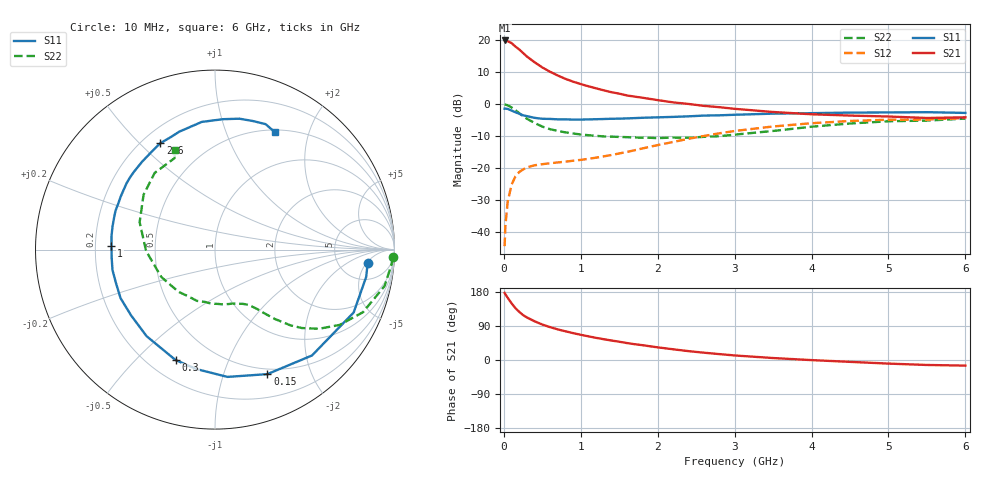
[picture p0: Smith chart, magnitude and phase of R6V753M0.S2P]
! SIEMENS Small Signal Semiconductors
! BFR193
! Si NPN RF Bipolar Junction Transistor in SOT23
! VCE = 0.75 V  IC = 3 mA
! Common Emitter S-Parameters:  May  1996
# GHz  S  MA  R  50
!  f  S11  S21  S12  S22
! GHz  MAG  ANG  MAG  ANG  MAG  ANG  MAG  ANG
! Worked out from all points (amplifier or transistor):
!   36 points, 10 MHz to 6 GHz, reference 50 ohm
!   highest |S21| = 19.9 dB at 10 MHz (marker M1)
!   |S21| within 3 dB of that: start of sweep to 208.3 MHz
!   unconditionally stable (mu >= 1): 1.001 GHz to 2.284 GHz; 5.435 GHz to end of sweep
!   at 250 MHz: K = 0.32, MSG = 18.2 dB, |S12| = -20.3 dB
!   at 1.4 GHz: K = 1.11, MAG = 7.8 dB, |S12| = -15.8 dB
!   at 6 GHz: K = 1.00, MAG = -0.3 dB, |S12| = -4.3 dB
!   S11 on the Smith chart (normalised r, x): 10 MHz: 10, -5; 150 MHz: 0.44, -1.41; 300 MHz: 0.31, -0.66; 1 GHz: 0.27, +0.02; 2.6 GHz: 0.27, +0.58; 6 GHz: 0.53, +1.50
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0.01  0.8537 -5.2  9.929 177.1  0.0061 86.2  0.9927 -2.5
0.02  0.856 -10.2  9.761 173.5  0.0127 84.5  0.9866 -4.9
0.05  0.8483 -24.4  9.649 164.2  0.0301 77.0  0.9665 -12.1
0.1  0.8 -47.5  9.049 149.8  0.0555 66.1  0.8955 -22.9
0.15  0.7526 -67.2  7.979 137.0  0.0746 56.7  0.8121 -31.1
0.2  0.7127 -84.4  7.177 127.0  0.0876 49.8  0.7281 -37.3
0.25  0.6737 -98.7  6.331 118.5  0.0963 44.6  0.6519 -42.1
0.3  0.6536 -109.6  5.572 112.2  0.1033 41.3  0.5956 -45.1
0.4  0.6148 -128.3  4.533 102.1  0.1118 36.8  0.5107 -49.2
0.5  0.5941 -141.9  3.766 93.6  0.1163 35.0  0.4489 -52.2
0.6  0.5917 -152.8  3.225 86.8  0.1201 34.7  0.4091 -54.4
0.7  0.5823 -161.4  2.822 80.8  0.1238 34.9  0.3845 -56.4
0.8  0.5824 -168.8  2.498 75.8  0.1272 35.7  0.3646 -58.5
1  0.5774 177.8  2.069 66.5  0.1356 39.3  0.3381 -63.3
1.1  0.5816 172.4  1.91 62.4  0.141 41.3  0.3294 -66.4
1.6  0.6026 150.7  1.375 44.7  0.1804 49.1  0.307 -83.1
2.2  0.6361 129.7  1.072 28.3  0.2582 51.1  0.3028 -109.4
2.6  0.6667 117.2  0.946 19.3  0.3202 47.9  0.3106 -130.7
3.5  0.7152 95.9  0.759 5.2  0.4509 33.6  0.3839 -178.8
4.5  0.742 79.4  0.667 -4.9  0.5491 16.0  0.5016 142.5
5.5  0.7537 68.0  0.612 -13.1  0.5792 -0.2  0.557 113.9
6  0.7339 62.9  0.627 -14.8  0.6107 -4.9  0.5985 111.8
